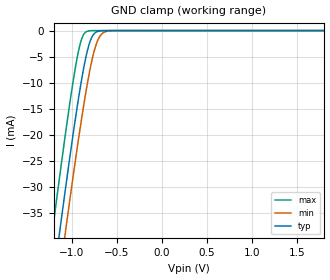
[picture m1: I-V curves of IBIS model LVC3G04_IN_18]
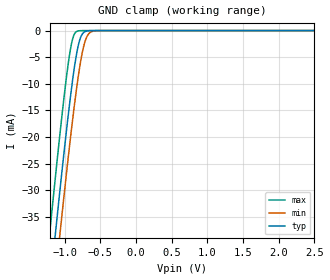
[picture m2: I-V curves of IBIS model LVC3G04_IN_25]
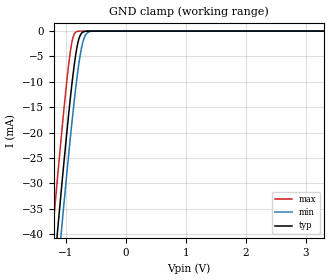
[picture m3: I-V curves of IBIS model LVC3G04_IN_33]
| TEXAS INSTRUMENTS INCORPORATED
| Standard Linear and Logic Group
| IBIS Model of SN74LVC3G04
| TRIPLE INVERTER GATE
| This file contains package information for the following:
|  SSOP 8-pin (DCT) package as [Component] LVC3G04_DCT
|  VSSOP 8-pin (DCU) package as [Component] LVC3G04_DCU
|  NanoStar WCSP 8-pin (YEA) package as [Component] LVC3G04_YEA
|  NanoFree WCSP 8-pin (YZA) package as [Component] LVC3G04_YZA
|  NanoStar WCSP 8-pin (YEP) package as [Component] LVC3G04_YEP
|  NanoFree WCSP 8-pin (YZP) package as [Component] LVC3G04_YZP
| This device can be powered at the following Vccs:
|  1.8 volt Vcc
|  2.5 volt Vcc
|  3.3 volt Vcc
|  5 volt Vcc
| This file provides unique models under the [Model Selector] for each Vcc.
| For operation at a specific Vcc, select the appropriate model after each
| [Model Selector] keyword.
[IBIS Ver]   3.2
[Comment char]  |_char
[File Name]   sn74lvc3g04.ibs
[File Rev]   1.2 | d_die
[Date]   May 18, 2004
[Source]   Data created from TI-SPICE simulations at TI-SLL.
[Notes]   The following is an IBIS list for the SN74LVC3G04.
   Please contact sllibis@ti.com with questions and
   comments concerning SLL IBIS models.
   - FILE REV HISTORY
   - 1.2 YEP and YZP packages added on 05/18/04
   - Power clamp data has been deleted since there is no
   power clamp diode in the device.
   - Due to the fact that the Device is 5.5-V Input tolarent,
   the pulldown model has some Non-Monotonic Warnings.
   - C_comp values are taken at a different test condition than
   the Ci in data sheet.
[Disclaimer] Property of Texas Instruments Incorporated. Unauthorized
   reproduction and/or distribution is strictly prohibited.
   This product is protected under copyright law.
   Created 2002, (C) Copyright  2002, Texas Instruments
   Incorporated, All Rights Reserved
   UNLESS THERE IS A SIGNED, WRITTEN AGREEMENT TO THE
   CONTRARY, TEXAS INSTRUMENTS (TI) IS PROVIDING THE IBIS
   MODELS AND WITHOUT ANY WARRANTY, EXPRESSED OR
   IMPLIED. TI assumes no liability for:
   1) the accuracy of the IBIS models provided to your
   company;
   2) the proper functioning of these IBIS Models in your
   design or for any resulting applications; or
   3) infringement of patents, copyrights or intellectual
   property rights resulting from your use of these IBIS
   models.
   TI provides IBIS Models as a service to our customers.
   You and your company shall not distribute, sell or give
   these models to anyone else without prior written
   permission from TI.
   TI reserves the right to make changes to our products or
   to discontinue any semiconductor product or service
   without notice, and advises our customers to obtain the
   latest version of relevant information to verify, before
   placing orders, that the information being relied on is
   current.
   Please be aware that your receipt and use of the IBIS
   information provided shall serve as acceptance of these
   terms and conditions. If you do not accept these terms,
   you should return or destroy the IBIS models and any
   other accompanying information immediately.
| Component LVC3G04_DCT 8-pin SSOP
[Component]   LVC3G04_DCT
[Manufacturer]   Texas Instruments, Inc.
[Package]
|   typ   min   max
R_pkg   2.900e-02   2.800e-02   3.100e-02
L_pkg   1.796e-09   1.666e-09   1.924e-09
C_pkg   1.090e-13   8.300e-14   1.360e-13
[Pin]   signal_name   model_name   R_pin   L_pin   C_pin
1   1A   LVC3G04_IN   3.100e-02   1.894e-09   1.340e-13
2   3Y   LVC3G04_OUT   2.800e-02   1.697e-09   8.600e-14
3   2A   LVC3G04_IN   3.000e-02   1.722e-09   8.600e-14
4   GND   GND   3.000e-02   1.861e-09   1.300e-13
5   2Y   LVC3G04_OUT   2.800e-02   1.924e-09   1.360e-13
6   3A   LVC3G04_IN   2.900e-02   1.736e-09   8.600e-14
7   1Y   LVC3G04_OUT   2.800e-02   1.666e-09   8.300e-14
8   VCC   POWER   3.000e-02   1.871e-09   1.320e-13
| Component LVC3G04_DCU 8-pin VSSOP
[Component]   LVC3G04_DCU
[Manufacturer]   Texas Instruments, Inc.
[Package]
|   typ   min   max
R_pkg   2.600e-02   2.300e-02   3.800e-02
L_pkg   1.394e-09   1.066e-09   2.046e-09
C_pkg   2.590e-13   2.150e-13   3.720e-13
[Pin]   signal_name   model_name   R_pin   L_pin   C_pin
1   1A   LVC3G04_IN   2.400e-02   1.520e-09   2.710e-13
2   3Y   LVC3G04_OUT   2.300e-02   1.112e-09   2.180e-13
3   2A   LVC3G04_IN   2.300e-02   1.070e-09   2.170e-13
4   GND   GND   2.700e-02   2.046e-09   3.720e-13
5   2Y   LVC3G04_OUT   2.700e-02   1.542e-09   2.730e-13
6   3A   LVC3G04_IN   2.300e-02   1.100e-09   2.240e-13
7   1Y   LVC3G04_OUT   2.300e-02   1.066e-09   2.150e-13
8   VCC   POWER   3.800e-02   1.696e-09   2.800e-13
| Component LVC3G04_YEA 8-pin NanoStar WCSP
[Component]   LVC3G04_YEA
[Manufacturer]   Texas Instruments, Inc.
[Package]
|   typ   min   max
R_pkg   0.001   0.001   0.001
L_pkg   0.021nH   0.021nH   0.021nH
C_pkg   0.043pF   0.042pF   0.044pF
[Pin]   signal_name   model_name   R_pin   L_pin   C_pin
1   1A   LVC3G04_IN   0.046   2.861nH   0.321pF
2   3Y   LVC3G04_OUT   0.037   2.437nH   0.286pF
3   2A   LVC3G04_IN   0.034   2.419nH   0.286pF
4   GND   GND   0.043   2.784nH   0.321pF
5   2Y   LVC3G04_OUT   0.043   2.784nH   0.321pF
6   3A   LVC3G04_IN   0.035   2.420nH   0.286pF
7   1Y   LVC3G04_OUT   0.037   2.437nH   0.286pF
8   VCC   POWER   0.046   2.860nH   0.321pF
| Component LVC3G04_YZA 8-pin NanoFree WCSP
[Component]   LVC3G04_YZA
[Manufacturer]   Texas Instruments, Inc.
[Package]
|   typ   min   max
R_pkg   0.001   0.001   0.001
L_pkg   0.021nH   0.021nH   0.021nH
C_pkg   0.043pF   0.042pF   0.044pF
[Pin]   signal_name   model_name   R_pin   L_pin   C_pin
1   1A   LVC3G04_IN   0.046   2.861nH   0.321pF
2   3Y   LVC3G04_OUT   0.037   2.437nH   0.286pF
3   2A   LVC3G04_IN   0.034   2.419nH   0.286pF
4   GND   GND   0.043   2.784nH   0.321pF
5   2Y   LVC3G04_OUT   0.043   2.784nH   0.321pF
6   3A   LVC3G04_IN   0.035   2.420nH   0.286pF
7   1Y   LVC3G04_OUT   0.037   2.437nH   0.286pF
8   VCC   POWER   0.046   2.860nH   0.321pF
| Component LVC3G04_YEP 8-pin DSBGA
[Component]   LVC3G04_YEP
[Manufacturer]   Texas Instruments, Inc.
[Package]
|   typ   min   max
R_pkg   1.000e-03   1.000e-03   1.000e-03
L_pkg   2.450e-11   2.400e-11   2.500e-11
C_pkg   6.550e-14   6.400e-14   6.700e-14
[Pin]   signal_name   model_name   R_pin   L_pin   C_pin
1   1A   LVC3G04_IN   1.000e-03   2.500e-11   6.400e-14
2   3Y   LVC3G04_OUT   1.000e-03   2.400e-11   6.700e-14
3   2A   LVC3G04_IN   1.000e-03   2.400e-11   6.700e-14
4   GND   GND   1.000e-03   2.500e-11   6.400e-14
5   2Y   LVC3G04_OUT   1.000e-03   2.500e-11   6.400e-14
6   3A   LVC3G04_IN   1.000e-03   2.400e-11   6.700e-14
7   1Y   LVC3G04_OUT   1.000e-03   2.400e-11   6.700e-14
8   VCC   POWER   1.000e-03   2.500e-11   6.400e-14
| Component LVC3G04_YZP 8-pin DSBGA
[Component]   LVC3G04_YZP
[Manufacturer]   Texas Instruments, Inc.
[Package]
|   typ   min   max
R_pkg   1.000e-03   1.000e-03   1.000e-03
L_pkg   2.450e-11   2.400e-11   2.500e-11
C_pkg   6.550e-14   6.400e-14   6.700e-14
[Pin]   signal_name   model_name   R_pin   L_pin   C_pin
1   1A   LVC3G04_IN   1.000e-03   2.500e-11   6.400e-14
2   3Y   LVC3G04_OUT   1.000e-03   2.400e-11   6.700e-14
3   2A   LVC3G04_IN   1.000e-03   2.400e-11   6.700e-14
4   GND   GND   1.000e-03   2.500e-11   6.400e-14
5   2Y   LVC3G04_OUT   1.000e-03   2.500e-11   6.400e-14
6   3A   LVC3G04_IN   1.000e-03   2.400e-11   6.700e-14
7   1Y   LVC3G04_OUT   1.000e-03   2.400e-11   6.700e-14
8   VCC   POWER   1.000e-03   2.500e-11   6.400e-14
| Model LVC3G04_IN
[Model Selector]   LVC3G04_IN
LVC3G04_IN_18   1.8 volt Vcc
LVC3G04_IN_25   2.5 volt Vcc
LVC3G04_IN_33   3.3 volt Vcc
LVC3G04_IN_50   5 volt Vcc
| Model LVC3G04_OUT
[Model Selector]   LVC3G04_OUT
LVC3G04_OUT_18   1.8 volt Vcc
LVC3G04_OUT_25   2.5 volt Vcc
LVC3G04_OUT_33   3.3 volt Vcc
LVC3G04_OUT_50   5 volt Vcc
| Models and submodels in the file (8): LVC3G04_IN_18 (Input), LVC3G04_IN_25 (Input), LVC3G04_IN_33 (Input), LVC3G04_IN_50 (Input), LVC3G04_OUT_18 (Output), LVC3G04_OUT_25 (Output), LVC3G04_OUT_33 (Output), LVC3G04_OUT_50 (Output)
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[Model]   LVC3G04_IN_18
Model_type  Input
Vinl=0.5775
Vinh=1.2675
| variable   typ   min   max
C_comp   3.50pF   3.03pF   4.29pF
[Temperature Range]   40   100   -40
| Ambient temperature   25   85   -40
[Voltage range]   1.8   1.65   1.95
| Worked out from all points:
|   GND clamp passes 1 mA (typ) near -0.77 V on its own axis
[GND Clamp]
| LVC3G04_IN_18
|   Voltage   I(typ)   I(min)   I(max)
-5V       -583.8mA   -590.8mA   -575.1mA
-1.21V    -48.93mA   -57.22mA   -38.3mA
-1.135V   -39.07mA   -47.36mA   -28.42mA
-1.075V   -31.35mA   -39.6mA    -20.75mA
-1.06V    -29.44mA   -37.69mA   -18.89mA
-960mV    -17.26mA   -25.26mA   -7.377mA
-885mV    -9.098mA   -16.55mA   -1.486mA
-830mV    -4.281mA   -10.75mA   -171.6uA
-780mV    -1.472mA   -6.227mA   -17.15uA
-715mV    -205.4uA   -2.128mA   -808.5nA
-650mV    -22.01uA   -443.9uA   -37.93nA
1.8V      3.326pA    6.142pA    3.026pA
[Model]   LVC3G04_IN_25
Model_type  Input
Vinl=0.7
Vinh=1.7
| variable   typ   min   max
C_comp   3.42pF   2.82pF   4.36pF
[Temperature Range]   40   100   -40
| Ambient temperature   25   85   -40
[Voltage range]   2.5   2.3   2.7
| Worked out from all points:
|   GND clamp passes 1 mA (typ) near -0.77 V on its own axis
[GND Clamp]
| LVC3G04_IN_25
|   Voltage   I(typ)   I(min)   I(max)
-5V       -583.8mA   -590.8mA   -575.1mA
-1.205V   -48.27mA   -56.56mA   -37.63mA
-1.13V    -38.42mA   -46.71mA   -27.77mA
-1.07V    -30.71mA   -38.96mA   -20.13mA
-1.05V    -28.19mA   -36.42mA   -17.65mA
-955mV    -16.68mA   -24.66mA   -6.874mA
-885mV    -9.098mA   -16.55mA   -1.486mA
-830mV    -4.281mA   -10.75mA   -171.6uA
-780mV    -1.472mA   -6.227mA   -17.15uA
-710mV    -173.7uA   -1.918mA   -639nA
-645mV    -18.49uA   -387.7uA   -29.98nA
2.5V      4.713pA    7.577pA    4.389pA
[Model]   LVC3G04_IN_33
Model_type  Input
Vinl=0.8
Vinh=2.0
| variable   typ   min   max
C_comp   3.35pF   2.67pF   4.39pF
[Temperature Range]   40   100   -40
| Ambient temperature   25   85   -40
[Voltage range]   3.3   3   3.6
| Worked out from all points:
|   GND clamp passes 1 mA (typ) near -0.77 V on its own axis
[GND Clamp]
| LVC3G04_IN_33
|   Voltage   I(typ)   I(min)   I(max)
-5V       -583.8mA   -590.8mA   -575.1mA
-1.215V   -49.6mA    -57.88mA   -38.96mA
-1.14V    -39.72mA   -48.01mA   -29.07mA
-1.08V    -31.98mA   -40.25mA   -21.38mA
-1.06V    -29.44mA   -37.69mA   -18.89mA
-925mV    -13.29mA   -21.11mA   -4.122mA
-875mV    -8.124mA   -15.45mA   -1.065mA
-820mV    -3.579mA   -9.774mA   -109.4uA
-770mV    -1.128mA   -5.445mA   -10.73uA
-715mV    -205.4uA   -2.128mA   -808.5nA
-590mV    -2.7uA     -81.86uA   -2.255nA
3.3V      6.304pA    9.258pA    5.93pA
